FUNCTION_BLOCK FB_DO_IED_LD1_LEDGGIO2_SPCSO1 EXTENDS FB_AcsiCommonControllableDataClass
VAR_INPUT
	stVal: FB_AcsiBATypeBOOLEAN := (fc:=ACSI_FC_ST, TrgOp:=ACSI_TrgOp_dchg, bLinkResult:=THIS^.AddDataToContainer(ipData:=stVal));
	q: FB_AcsiDATypeQuality := (fc:=ACSI_FC_ST, TrgOp:=ACSI_TrgOp_qchg, bLinkResult:=THIS^.AddDataToContainer(ipData:=q));
	t: FB_AcsiDATypeTimeStamp := (fc:=ACSI_FC_ST, bLinkResult:=THIS^.AddDataToContainer(ipData:=t));
	stSeld: FB_AcsiBATypeBOOLEAN := (fc:=ACSI_FC_ST, TrgOp:=ACSI_TrgOp_dchg, bLinkResult:=THIS^.AddDataToContainer(ipData:=stSeld));
	ctlModel: FB_AcsiDATypeCtlModels := (fc:=ACSI_FC_CF, TrgOp:=ACSI_TrgOp_dchg, eValue:=E_AcsiCtlModels.DirectWithNormalSecurity, bLinkResult:=THIS^.AddDataToContainer(ipData:=ctlModel));
	Oper: FB_AcsiCDC_Oper_BOOLEAN := (fc:=ACSI_FC_CO, bLinkResult:=THIS^.AddDataToContainer(ipData:=Oper));
END_VAR
VAR
END_VAR

END_FUNCTION_BLOCK
